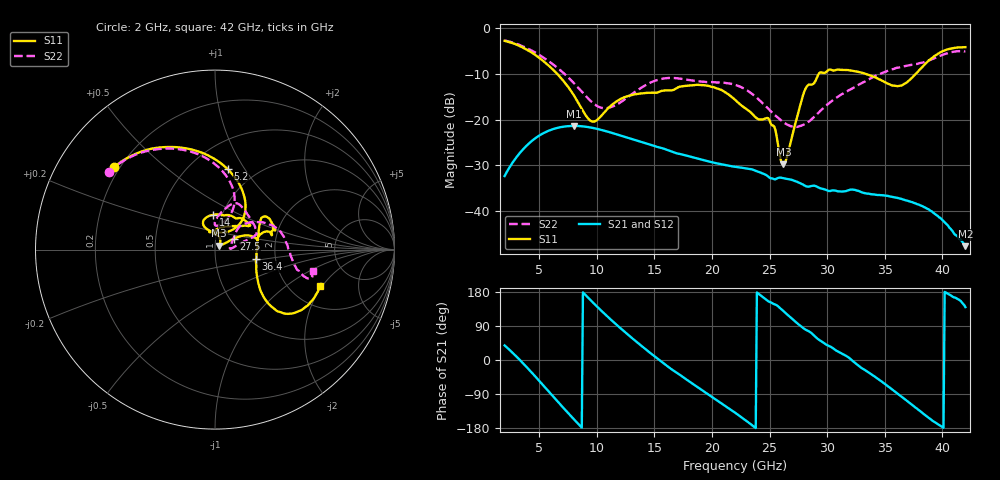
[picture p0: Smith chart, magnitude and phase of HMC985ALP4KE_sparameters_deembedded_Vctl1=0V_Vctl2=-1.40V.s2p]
!s2p File: Measurements: S11, S21, S12, S22
# GHz S dB R 50.0
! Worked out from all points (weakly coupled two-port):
!   401 points, 2 GHz to 42 GHz, reference 50 ohm
!   highest |S21| = -21.37 dB at 8 GHz (marker M1); lowest = -47.7 dB at 42 GHz (marker M2)
!   lowest |S11| = -29.8 dB at 26.2 GHz (marker M3), VSWR 1.07, Z = 52.4 + j2.3 ohm
!   |S11| at or under -10 dB: 6.566 GHz to 29.27 GHz (22.7 GHz wide, 127 % of centre); 33.35 GHz to 37.69 GHz (4.34 GHz wide, 12.2 % of centre)
!   |S22| runs from -21.6 to -2.7 dB; largest |S21 - S12| = 0.00015
!   S11 on the Smith chart (normalised r, x): 2 GHz: 0.18, +0.35; 5.2 GHz: 0.75, +0.84; 14 GHz: 0.91, +0.37; 27.5 GHz: 1.22, +0.15; 36.4 GHz: 1.58, -0.18; 42 GHz: 2.91, -1.91
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2  -2.76 140.7  -32.35 38.5  -32.35 38.5  -2.68 143.8
3.5  -4.13 113.1  -26.78 -5.4  -26.79 -5.5  -3.88 118.8
5.2  -6.86 81.1  -23.20 -61.6  -23.20 -61.7  -6.14 92.6
8  -14.64 46.1  -21.37 -156.0  -21.38 -156.0  -11.97 66.1
8.7  -17.66 51.9  -21.46 -178.4  -21.46 -178.4  -13.89 66.7
9.7  -20.45 84.7  -21.84 150.6  -21.84 150.6  -16.44 74.9
10.8  -18.01 112.3  -22.52 118.3  -22.53 118.3  -17.50 87.2
14  -14.23 92.5  -24.96 34.3  -24.96 34.3  -12.81 77.1
15.4  -13.94 73.0  -26.06 0.9  -26.07 0.9  -11.22 68.6
19.4  -12.52 34.5  -28.96 -85.1  -28.96 -85.1  -11.74 37.4
22  -15.63 52.3  -30.31 -138.9  -30.32 -138.9  -12.39 19.7
25  -20.16 98.1  -32.70 153.2  -32.71 153.2  -17.91 11.5
26.2  -29.78 42.5  -32.80 128.8  -32.81 128.8  -20.56 4.4
27.5  -18.38 29.9  -33.73 94.5  -33.74 94.3  -21.50 6.8
28.1  -13.35 20.8  -34.48 80.7  -34.52 80.5  -20.94 14.3
28.7  -12.30 12.9  -34.48 69.2  -34.47 69.4  -19.80 22.7
31  -9.07 23.3  -35.69 21.4  -35.72 21.4  -14.86 43.0
33.3  -9.95 34.4  -36.09 -26.9  -36.12 -27.0  -11.63 35.5
35.4  -12.27 12.3  -36.78 -72.2  -36.78 -72.2  -9.21 22.7
36.4  -12.57 -12.9  -37.31 -95.7  -37.34 -95.6  -8.44 15.3
39.5  -5.80 -43.3  -40.91 -167.2  -40.82 -167.0  -6.34 -14.3
42  -4.15 -19.0  -47.69 139.5  -47.70 139.9  -5.07 -12.6
